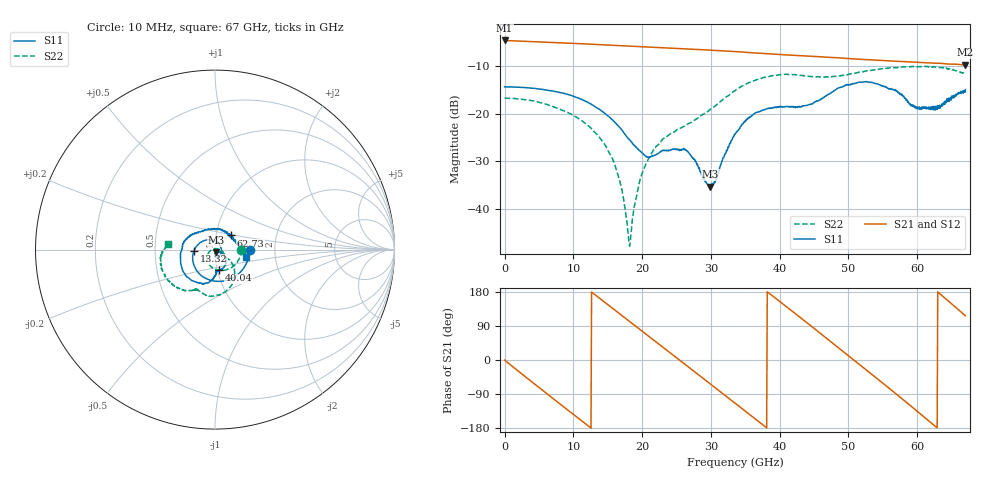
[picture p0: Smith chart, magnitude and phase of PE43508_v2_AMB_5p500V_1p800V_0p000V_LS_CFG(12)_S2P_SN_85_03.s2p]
!Keysight Technologies,N5227A,US51270237,A.10.43.00
!Date: Wednesday, August 22, 2018 17:07:46
!Correction: S11(Full 2 Port(1,3))
!S31(Full 2 Port(1,3))
!S13(Full 2 Port(1,3))
!S33(Full 2 Port(1,3))
!S2P File: Measurements: S11, S31, S13, S33:
# Hz S  dB  R 50
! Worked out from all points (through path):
!   801 points, 10 MHz to 67 GHz, reference 50 ohm
!   highest |S21| = -4.53 dB at 10 MHz (marker M1); lowest = -9.7 dB at 66.92 GHz (marker M2)
!   group delay of S21, straight-line fit = 39.5 ps
!   lowest |S11| = -35.3 dB at 29.9 GHz (marker M3), VSWR 1.03, Z = 50.7 - j1.57 ohm
!   |S11| at or under -10 dB: start of sweep to end of sweep
!   |S22| runs from -47.9 to -10.0 dB; largest |S21 - S12| = 0.0031
!   S11 on the Smith chart (normalised r, x): 10 MHz: 1.48, -0.00; 13.32 GHz: 0.79, -0.01; 40.04 GHz: 1.02, -0.24; 62.73 GHz: 1.18, +0.19; 67 GHz: 1.42, -0.13
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1e7  -14.29 -0.4  -4.53 -0.2  -4.53 -0.2  -16.71 -0.4
2.522125e9  -14.43 -36.1  -4.68 -37.0  -4.68 -36.9  -16.92 -28.4
5.70415e9  -14.89 -78.9  -4.87 -82.5  -4.87 -82.4  -17.82 -62.1
8.216275e9  -15.54 -111.6  -5.04 -118.2  -5.03 -118.1  -19.13 -87.4
1.123082e10  -16.99 -149.3  -5.23 -160.7  -5.22 -160.7  -21.42 -115.9
1.332426e10  -18.63 -176.5  -5.37 169.8  -5.36 169.8  -24.17 -135.4
1.617134e10  -22.00 141.8  -5.57 129.8  -5.56 129.8  -31.34 -165.6
1.818104e10  -25.55 101.9  -5.71 101.6  -5.70 101.6  -47.92 91.3
1.985579e10  -28.06 58.2  -5.83 78.1  -5.83 78.1  -33.14 5.4
2.236791e10  -28.32 -18.4  -6.02 42.9  -6.02 42.9  -26.43 -18.6
2.638731e10  -27.75 -84.4  -6.31 -13.4  -6.30 -13.4  -22.35 -35.3
2.990429e10  -35.34 -64.7  -6.57 -63.0  -6.56 -63.0  -19.11 -37.1
3.3505e10  -24.37 -32.9  -6.87 -113.9  -6.87 -113.9  -15.10 -51.1
3.68545e10  -19.65 -56.5  -7.20 -161.1  -7.20 -161.1  -12.73 -71.2
4.003652e10  -18.57 -79.1  -7.50 154.0  -7.49 154.0  -11.77 -91.0
4.472582e10  -17.91 -87.0  -7.86 87.4  -7.85 87.4  -12.16 -110.8
5.033624e10  -13.75 -114.6  -8.38 6.6  -8.38 6.5  -11.58 -119.8
5.586291e10  -14.78 178.6  -8.82 -73.8  -8.82 -74.1  -10.33 -138.6
5.89612e10  -17.88 126.0  -9.07 -119.7  -9.07 -119.9  -10.08 -150.5
6.272939e10  -18.40 41.0  -9.34 -176.5  -9.37 -176.7  -10.14 -167.3
6.691626e10  -15.47 -12.8  -9.67 118.0  -9.73 118.2  -11.43 174.2
6.7e10  -14.89 -14.1  -9.66 116.6  -9.72 116.8  -11.51 173.1
